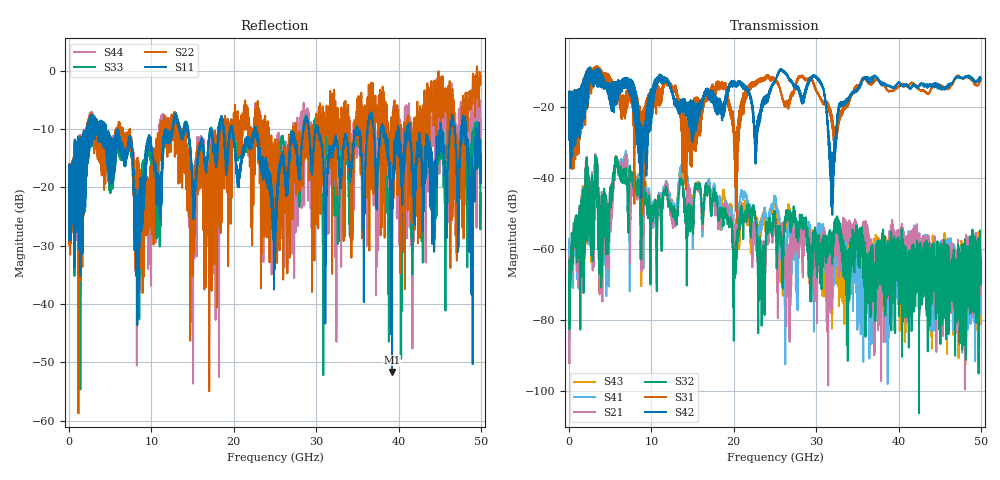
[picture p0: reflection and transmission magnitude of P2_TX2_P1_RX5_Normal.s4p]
!Keysight Technologies,N5225B,MY57041031,A.13.20.10
!Date: Friday, May 31, 2019 11:21:31
!Correction: S11(Full 4 Port(1,2,3,4))
!S12(Full 4 Port(1,2,3,4))
!S13(Full 4 Port(1,2,3,4))
!S14(Full 4 Port(1,2,3,4))
!S21(Full 4 Port(1,2,3,4))
!S22(Full 4 Port(1,2,3,4))
!S23(Full 4 Port(1,2,3,4))
!S24(Full 4 Port(1,2,3,4))
!S31(Full 4 Port(1,2,3,4))
!S32(Full 4 Port(1,2,3,4))
!S33(Full 4 Port(1,2,3,4))
!S34(Full 4 Port(1,2,3,4))
!S41(Full 4 Port(1,2,3,4))
!S42(Full 4 Port(1,2,3,4))
!S43(Full 4 Port(1,2,3,4))
!S44(Full 4 Port(1,2,3,4))
!S4P File: Measurements: <S11,S12,S13,S14>,
!<S21,S22,S23,S24>,
!<S31,S32,S33,S34>,
!<S41,S42,S43,S44>:
# Hz S  dB  R 50.0
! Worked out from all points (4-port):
!   5000 points, 10 MHz to 50 GHz, reference 50 ohm
!   strongest paths, dB at 10 MHz, 12.51 GHz, 25.01 GHz, 37.51 GHz, 50 GHz:
!     S42: -19.5, -15.6, -13.0, -12.0, -12.1
!     S31: -19.3, -14.8, -13.0, -12.4, -12.6
!     S32: -63.8, -48.6, -50.8, -58.1, -66.2
!     S21: -62.2, -51.0, -53.5, -82.3, -67.6
!     S41: -57.3, -47.8, -45.6, -65.0, -60.9
!     S43: -65.6, -47.2, -46.1, -62.4, -65.0
!   lowest |S11| = -51.7 dB at 39.22 GHz (marker M1), VSWR 1.01, Z = 49.8 + j0.209 ohm
!   |S11| at or under -10 dB: 4.481 GHz to 11.72 GHz (7.238 GHz wide, 89.4 % of centre); 22.73 GHz to 28.47 GHz (5.745 GHz wide, 22.4 % of centre); 30.26 GHz to 34.82 GHz (4.561 GHz wide, 14 % of centre)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
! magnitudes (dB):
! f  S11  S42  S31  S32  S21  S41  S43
! 10 MHz  -19.2  -19.5  -19.3  -63.8  -62.2  -57.3  -65.6
! 6.84 GHz  -15.4  -14.5  -22.2  -37.9  -34.6  -33.3  -35.5
! 8.72 GHz  -21.2  -30.6  -25.6  -58.7  -51.9  -45.8  -53.7
! 29.85 GHz  -11.2  -11.5  -14.3  -58.1  -63.1  -70.1  -64.7
! 31.94 GHz  -13.3  -35.9  -25.3  -58.2  -65.0  -64.0  -62.7
! 39.22 GHz  -51.7  -14.5  -15.6  -73.6  -59.8  -76.6  -61.6
! 50 GHz  -14.4  -12.1  -12.6  -66.2  -67.6  -60.9  -65.0
